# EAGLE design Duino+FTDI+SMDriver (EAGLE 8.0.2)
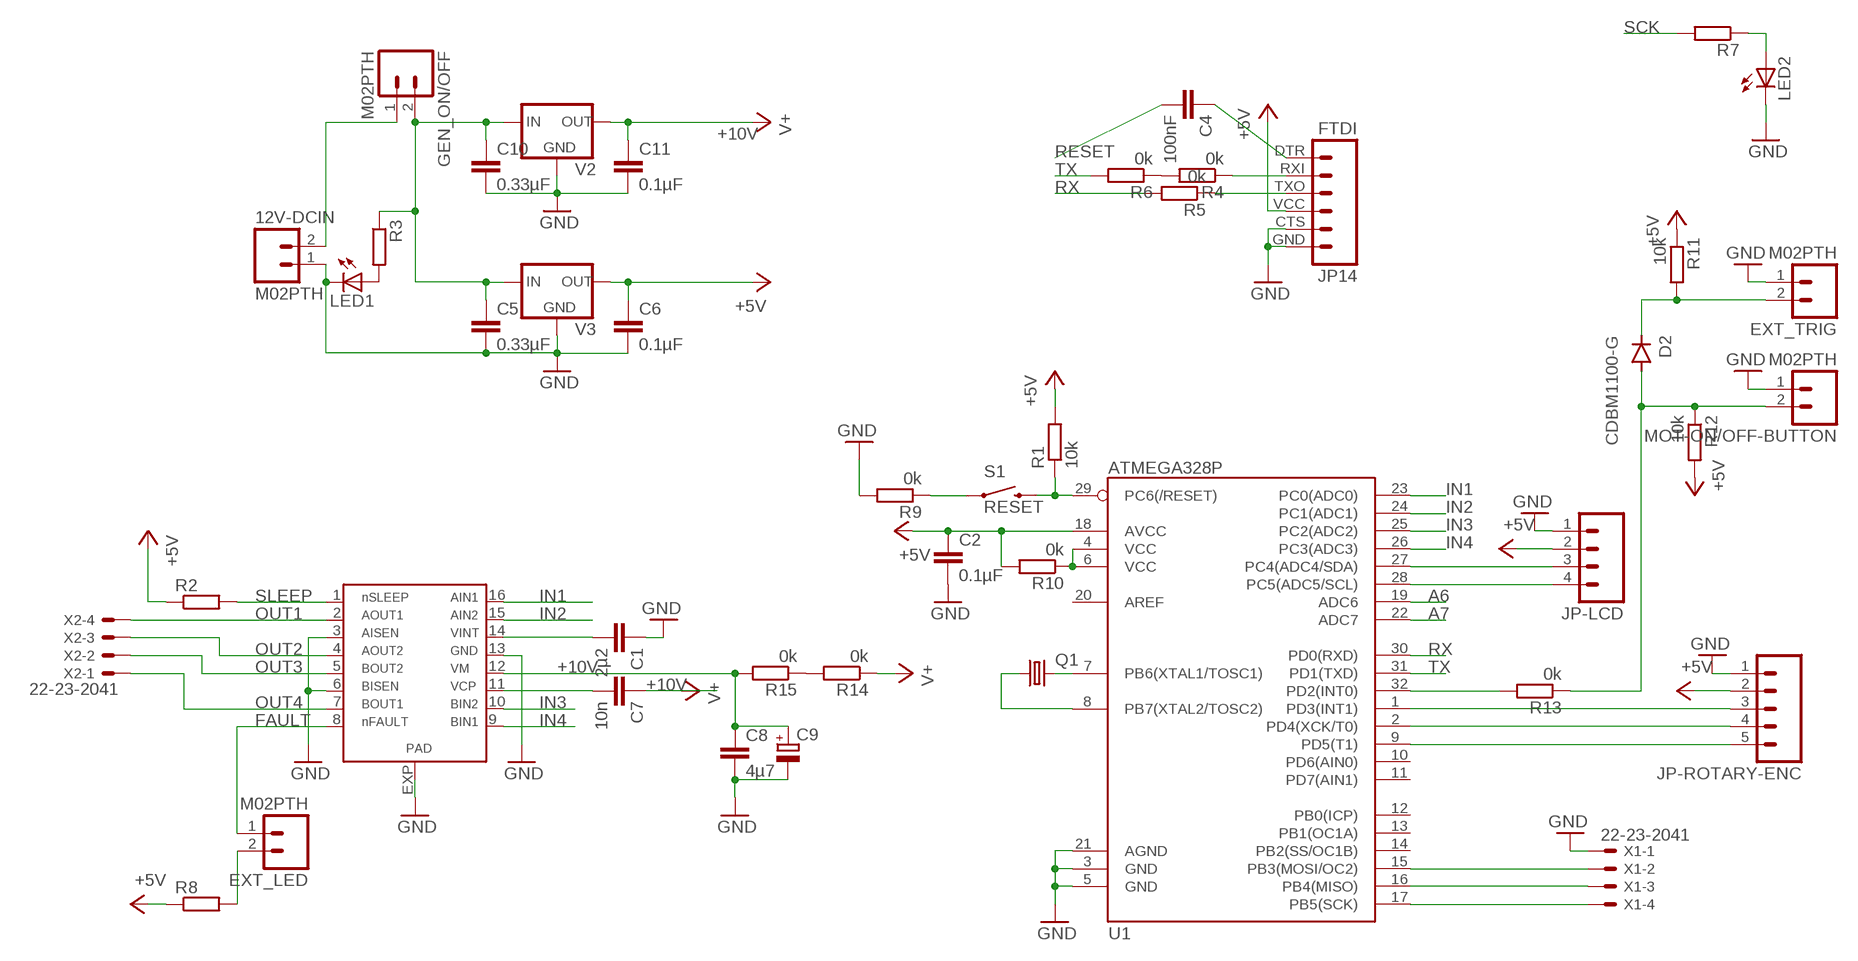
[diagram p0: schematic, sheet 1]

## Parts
12V-DCIN  M02PTH  [1X02]
C1  2µ2  C-EUC1206  [C1206]
C2  0.1µF  C-EUC1206  [C1206]
C4  100nF  C-EUC1206  [C1206]
C5  0.33µF  C-EUC1206  [C1206]
C6  0.1µF  C-EUC1206  [C1206]
C7  10n  C-EUC1206  [C1206]
C8  4µ7  C-EUC1206  [C1206]
C9  CPOL-EU153CLV-0605  [153CLV-0605]
C10  0.33µF  C-EUC1206  [C1206]
C11  0.1µF  C-EUC1206  [C1206]
D2  CDBM1100-G  [MINI-SMA]
EXT_LED  M02PTH  [1X02]
EXT_TRIG  M02PTH  [1X02]
GEN_ON/OFF  M02PTH  [1X02]
IC1  DRV8833  [HTSSOP16PWP]
JP14  FTDI  FTDI_BASICPTH  [FTDI_BASIC]
JP-LCD  M04PTH  [1X04]
JP-ROTARY-ENC  M05PTH  [1X05]
LED1  LEDSMT1206  [1206]
LED2  LEDSMT1206  [1206]
MOT-ON/OFF-BUTTON  M02PTH  [1X02]
Q1  CRYSTALSM49  [SM49]
R1  10k  R-EU_R1206  [R1206]
R2  R-EU_R1206  [R1206]
R3  R-EU_R1206  [R1206]
R4  0k  R-EU_R1206  [R1206]
R5  0k  R-EU_R1206  [R1206]
R6  0k  R-EU_R1206  [R1206]
R7  R-EU_R1206  [R1206]
R8  R-EU_R1206  [R1206]
R9  0k  R-EU_R1206  [R1206]
R10  0k  R-EU_R1206  [R1206]
R11  10k  R-EU_R1206  [R1206]
R12  10k  R-EU_R1206  [R1206]
R13  0k  R-EU_R1206  [R1206]
R14  0k  R-EU_R1206  [R1206]
R15  0k  R-EU_R1206  [R1206]
S1  RESET  SWITCH-MOMENTARY-2-SMD-1101NE  [TACTILE-SWITCH-1101NE]
U1  ATMEGA328P  ATMEGA328_SMT  [TQFP32-08]
V2  UA78XX  [D2PACK]
V3  UA78MXX  [DPACK]
X1  22-23-2041  [22-23-2041]
X2  22-23-2041  [22-23-2041]

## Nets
+5V: C2.1 C6.1 JP14.VCC JP-LCD.2 JP-ROTARY-ENC.2 R1.2 R2.1 R8.1 R10.1 R10.2 R11.1 R12.2 U1.4(VCC) U1.6(VCC) U1.18(AVCC) V3.OUT
+10V: C7.1 C8.1 C9.+ C11.1 IC1.12 R14.1 R15.2 V2.OUT ; supply symbol labelled V+
A4: JP-LCD.3 U1.27(PC4(ADC4/SDA))
A5: JP-LCD.4 U1.28(PC5(ADC5/SCL))
A6: U1.19(ADC6)
A7: U1.22(ADC7)
FAULT: EXT_LED.1 IC1.8
GND: 12V-DCIN.1 C1.1 C2.2 C5.2 C6.2 C8.2 C9.- C10.2 C11.2 EXT_TRIG.1 IC1.3 IC1.6 IC1.13 IC1.EXP JP14.CTS JP14.GND JP-LCD.1 JP-ROTARY-ENC.1 LED1.C LED2.C MOT-ON/OFF-BUTTON.1 R9.1 R9.2 S1.1 U1.3(GND) U1.5(GND) U1.21(AGND) V2.CASE(GND) V2.GND V3.CASE(GND) X1.1
IN1: IC1.16 U1.23(PC0(ADC0))
IN2: IC1.15 U1.24(PC1(ADC1))
IN3: IC1.10 U1.25(PC2(ADC2))
IN4: IC1.9 U1.26(PC3(ADC3))
N$1: Q1.2 U1.7(PB6(XTAL1/TOSC1))
N$2: Q1.1 U1.8(PB7(XTAL2/TOSC2))
N$3: JP-ROTARY-ENC.3 U1.1(PD3(INT1))
N$4: 12V-DCIN.2 GEN_ON/OFF.1
N$5: C4.1 JP14.DTR
N$6: JP14.RXI R4.1
N$7: JP14.TXO R5.1
N$8: R4.2 R6.1
N$9: LED2.A R7.1
N$10: R13.2 U1.32(PD2(INT0))
N$11: D2.KATHODE EXT_TRIG.2 R11.2
N$13: R14.2 R15.1
N$14: LED1.A R3.2
N$15: D2.ANODE MOT-ON/OFF-BUTTON.2 R12.1 R13.1
N$17: U1.16(PB4(MISO)) X1.3
N$18: U1.15(PB3(MOSI/OC2)) X1.2
N$19: JP-ROTARY-ENC.4 U1.2(PD4(XCK/T0))
N$20: JP-ROTARY-ENC.5 U1.9(PD5(T1))
N$22: C1.2 IC1.14
N$23: C7.2 IC1.11
N$25: EXT_LED.2 R8.2
N$26: C5.1 C10.1 GEN_ON/OFF.2 R3.1 V2.IN V3.IN
OUT1: IC1.2 X2.4
OUT2: IC1.4 X2.3
OUT3: IC1.5 X2.2
OUT4: IC1.7 X2.1
RESET: C4.2 R1.1 S1.2 U1.29(PC6(/RESET))
RX: R5.2 U1.30(PD0(RXD))
SCK: R7.2 U1.17(PB5(SCK)) X1.4
SLEEP: IC1.1 R2.2
TX: R6.2 U1.31(PD1(TXD))
Unconnected: U1.10(PD6(AIN0)) U1.11(PD7(AIN1)) U1.12(PB0(ICP)) U1.13(PB1(OC1A)) U1.14(PB2(SS/OC1B)) U1.20(AREF)

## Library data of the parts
12V-DCIN EXT_LED EXT_TRIG GEN_ON/OFF MOT-ON/OFF-BUTTON = SparkFun-Connectors:M02: Standard 2-pin 0.1" header. Use with
C1 C2 C4-C8 C10 C11 = rcl:C-EU: CAPACITOR, European symbol
C9 = rcl:CPOL-EU: POLARIZED CAPACITOR, European symbol
D2 = fab:CDBM1100-G: Diode schottky 100V 1A mini-SMA as found in the fablab inventory
IC1 = 1Axel:DRV8833
JP14 = SparkFun-Connectors:FTDI_BASIC: FTDI Basic header with labels
JP-LCD = SparkFun-Connectors:M04: Header 4 Standard 4-pin 0.1" header. Use with straight break away headers (SKU : PRT-00116), right angle break away headers (PRT-00553), swiss pins (PRT-00743), machine pins (PRT-00117), and female headers (PRT-00115). Molex polarized connector foot print use with SKU : PRT-08231 with associated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
JP-ROTARY-ENC = SparkFun-Connectors:M05: Header 5 Standard 5-pin 0.1" header. Use with straight break away headers (SKU : PRT-00116), right angle break away headers (PRT-00553), swiss pins (PRT-00743), machine pins (PRT-00117), and female headers (PRT-00115). Molex polarized connector foot print use with SKU : PRT-08230 with associated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
LED1 LED2 = led:LED: LED
Q1 = crystal:CRYSTAL: CRYSTAL; OC_FARNELL: unknown; OC_NEWARK: unknown
R1-R15 = rcl:R-EU_: RESISTOR, European symbol
S1 = SparkFun-Electromechanical:SWITCH-MOMENTARY-2: Various NO switches- pushbuttons, reed, etc
U1 = SparkFun-DigitalIC:ATMEGA328_SMT: 32-Pin Atmega328 part Commonly used on Arduino compatible boards Available in QFP and QFN packages TQFP is IC-09069 QFN is non-stock; PROD_ID: IC-09069
V2 = Power:UA78XX
V3 = Power:UA78MXX
X1 X2 = con-molex:22-23-2041: .100" (2.54mm) Center Header - 4 Pin; MF: MOLEX; MPN: 22-23-2041; OC_FARNELL: 1462920; OC_NEWARK: 38C0355

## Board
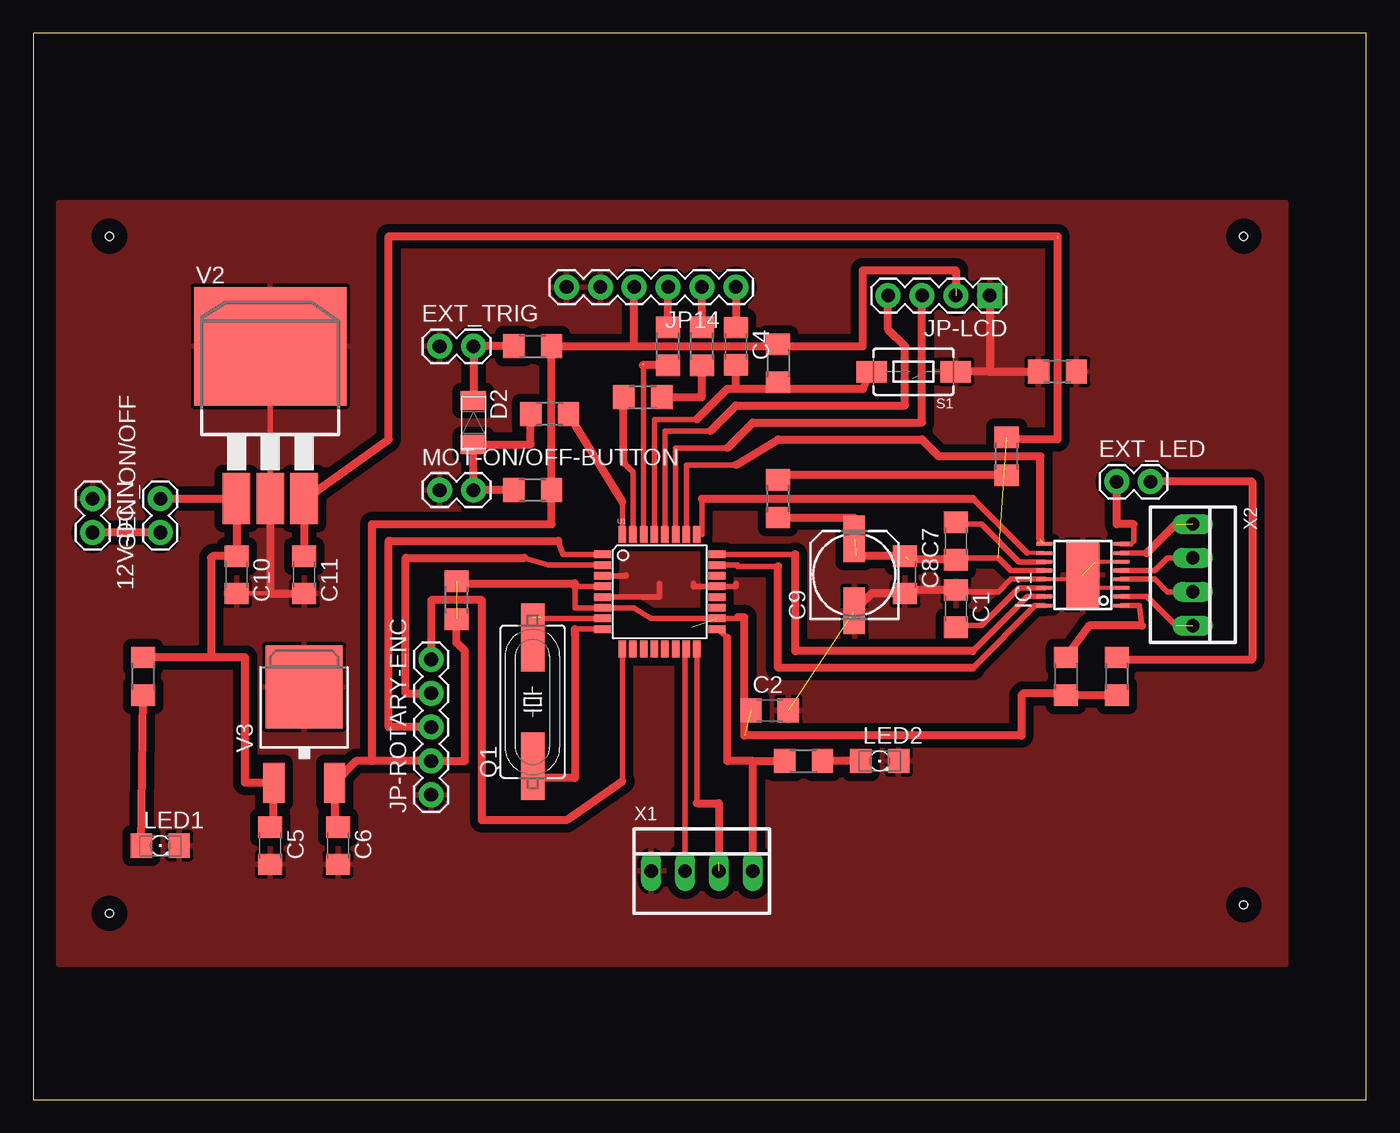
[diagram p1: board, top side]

Size 100 x 80 mm. Coordinates in mm from the lower left corner, seen from the top.
Outline: 0,0 100,0 100,80 0,80 0,0
Copper layers (1*16): Top 0.035mm / dielectric 1.5mm / Bottom 0.035mm
Design rules "default": minimum track width 10mil, minimum drill 24mil, track to track 8mil, track to pad 8mil, pad to pad 8mil, via to via 8mil, smd to smd 8mil, copper to edge 40mil, drill to drill 8mil, minimum pad ring 10mil, minimum via ring 8mil, stop-mask expansion 4mil, vias tented up to drill 0mil, thermal gap 10mil
Holes 0.6 mm at 5.71,13.97 5.71,64.77 90.81,64.77 90.81,14.61

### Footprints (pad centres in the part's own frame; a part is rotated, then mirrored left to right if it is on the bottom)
1X02 = drill 1.016 pad 1.88: 1 0,0; 2 2.54,0
C1206 = smd 1.6 x 1.8: 1 -1.4,0; 2 1.4,0
153CLV-0605 = smd 3.5 x 1.6: + 2.7,0; - -2.7,0
MINI-SMA = smd 1.4 x 1.9: ANODE 1.65,0; KATHODE -1.65,0
HTSSOP16PWP = smd 0.27 x 1.2: 1 -3.588,-2.9; 2 -2.895,-2.9; 3 -2.245,-2.9; 4 -1.595,-2.9; 5 -0.945,-2.9; 6 -0.295,-2.9; 7 0.355,-2.9; 8 1.048,-2.9; 9 1.048,2.9; 10 0.355,2.9; 11 -0.295,2.9; 12 -0.945,2.9; 13 -1.595,2.9; 14 -2.245,2.9; 15 -2.895,2.9; 16 -3.588,2.9 | smd 5.08 x 2.46: EXP -1.27,0
FTDI_BASIC = drill 1.016 pad 1.88: CTS 10.16,0; DTR 0,0; GND 12.7,0; RXI 2.54,0; TXO 5.08,0; VCC 7.62,0
1X04 = drill 1.016 pad 1.88 square: 1 0,0 | drill 1.016 pad 1.88: 2 2.54,0; 3 5.08,0; 4 7.62,0
1X05 = drill 1.016 pad 1.88: 1 0,0; 2 2.54,0; 3 5.08,0; 4 7.62,0; 5 10.16,0
1206 = smd 1.6 x 1.803: A -1.422,0; C 1.422,0
SM49 = smd 5.08 x 1.778: 1 -4.826,0; 2 4.826,0
R1206 = smd 1.6 x 1.803: 1 -1.422,0; 2 1.422,0
TACTILE-SWITCH-1101NE = smd 2.3 x 1.6: 1 -3.15,0; 2 3.15,0
TQFP32-08 = smd 1.27 x 0.559: 1 -4.293,2.8; 2 -4.293,2; 3 -4.293,1.2; 4 -4.293,0.4; 5 -4.293,-0.4; 6 -4.293,-1.2; 7 -4.293,-2; 8 -4.293,-2.8; 17 4.293,-2.8; 18 4.293,-2; 19 4.293,-1.2; 20 4.293,-0.4; 21 4.293,0.4; 22 4.293,1.2; 23 4.293,2; 24 4.293,2.8 | smd 0.559 x 1.27: 9 -2.8,-4.293; 10 -2,-4.293; 11 -1.2,-4.293; 12 -0.4,-4.293; 13 0.4,-4.293; 14 1.2,-4.293; 15 2,-4.293; 16 2.8,-4.293; 25 2.8,4.293; 26 2,4.293; 27 1.2,4.293; 28 0.4,4.293; 29 -0.4,4.293; 30 -1.2,4.293; 31 -2,4.293; 32 -2.8,4.293
D2PACK = smd 11.43 x 8.89: CASE 3.81,6.35 | smd 2.083 x 3.81: GND 3.81,-5.08; IN 1.27,-5.08; OUT 6.35,-5.08
DPACK = smd 5.8 x 6.2: CASE 0,2.38 | smd 1.6 x 3: IN -2.28,-4.8; OUT 2.28,-4.8
22-23-2041 = drill 1 long: 1 -3.81,0; 2 -1.27,0; 3 1.27,0; 4 3.81,0

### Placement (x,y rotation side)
12V-DCIN  4.45,45.09 270 top
C1  69.22,36.83 270 top
C2  55.24,29.21 0 top
C4  52.7,56.52 270 top
C5  17.78,19.05 270 top
C6  22.86,19.05 270 top
C7  69.22,41.91 90 top
C8  65.41,39.37 270 top
C9  61.59,39.37 90 top
C10  15.24,39.37 270 top
C11  20.32,39.37 270 top
D2  33.02,50.8 270 top
EXT_LED  81.28,46.35 0 top
EXT_TRIG  30.48,56.52 0 top
GEN_ON/OFF  9.53,42.55 90 top
IC1  78.74,40.64 90 top
JP14  52.7,60.96 180 top
JP-LCD  71.75,60.33 180 top
JP-ROTARY-ENC  29.84,22.86 90 top
LED1  9.53,19.05 0 top
LED2  63.5,25.4 0 top
MOT-ON/OFF-BUTTON  30.48,45.72 0 top
Q1  37.47,29.84 90 top
R1  55.88,55.24 90 top
R2  77.47,31.75 90 top
R3  8.26,31.75 270 top
R4  50.16,56.52 270 top
R5  47.62,56.52 270 top
R6  45.72,52.7 180 top
R7  57.78,25.4 180 top
R8  81.28,31.75 90 top
R9  76.83,54.61 0 top
R10  31.75,37.47 270 top
R11  37.47,56.52 180 top
R12  37.47,45.72 0 top
R13  38.73,51.44 0 top
R14  73.03,48.26 270 top
R15  55.88,45.09 270 top
S1  66.04,54.61 180 top
U1  46.99,38.1 0 top
V2  13.97,50.16 0 top
V3  20.32,28.57 0 top
X1  50.16,17.14 0 top
X2  87,39.37 270 top

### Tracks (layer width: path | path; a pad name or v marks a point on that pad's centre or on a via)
+5V  (5 unrouted)
  Top 0.305: 55.88,56.52 R1.2
  Top 0.406: 22.6,20.71 C6.1 | 52.84,36.2 52.84,36.1 U1.18 46.35,36.1 45.09,36.9 U1.6 40.64,36.9 40.64,38.5 U1.4
  Top 0.61: R8.1 R2.1 77.32,30.48 74.3,30.48 74.14,30.33 74.14,27.3 53.34,27.3 53.34,36.2 52.84,36.2 | 25.4,25.4 JP-ROTARY-ENC.2 32.38,25.4 32.38,33.66 31.75,34.29 R10.2 | 25.4,25.4 25.4,43.18 38.89,43.18 R12.2 R11.1 45.09,56.52 | 45.09,56.52 JP14.VCC | 45.09,56.52 55.88,56.52 62.23,56.52 62.23,62.23 69.22,62.23 69.22,60.85 | 40.64,38.5 40.64,38.73 31.75,38.73 | 22.6,20.71 V3.OUT 24.23,25.4 25.4,25.4
+10V  (4 unrouted)
  Top 0.305: C7.1 69.34,40.64 | C11.1 20.45,45.09 | 61.73,40.77 61.59,40.64
  Top 0.406: 69.34,40.64 72.39,40.64 73.33,39.7 IC1.12
  Top 0.61: C7.1 65.67,40.51 | V2.OUT C11.1 | 20.45,45.09 26.67,49.53 26.67,64.77 76.83,64.77 | 76.83,64.61 76.83,49.53 74.3,49.53 R14.1 | C8.1 61.73,40.77 | R15.2 61.59,43.66 C9.+
A4
  Top 0.406: 52.07,48.9 48.19,48.9 U1.27
  Top 0.61: JP-LCD.3 66.67,50.8 53.98,50.8 52.07,48.9
A5
  Top 0.406: 50.8,50.16 47.39,50.16 U1.28
  Top 0.61: 50.8,50.16 52.7,52.07 65.41,52.07 65.41,56.52 64.14,57.78 JP-LCD.4
FAULT
  Top 0.305: 82.33,41.69 82.55,41.91
  Top 0.406: IC1.8 82.33,41.69 | 82.55,41.91 82.55,43.18
  Top 0.61: 82.55,43.18 81.28,43.18 EXT_LED.1
GND  (2 unrouted)
  Top 0.305: 69.34,38.1 C1.1 | IC1.13 78.42,39.05 IC1.EXP | IC1.3 79.03,38.4 78.74,38.1 | IC1.6 79.67,40.34 79.38,40.64 | 65.67,38.23 C8.2 | 17.78,37.97 C10.2
  Top 0.406: 17.78,55.88 V2.GND | IC1.13 73.33,39.05 72.39,38.1 69.34,38.1 | 49.53,38.73 49.53,38.5 U1.21 52.7,38.5 52.7,38.73 | U1.3 44.45,39.3 44.45,39.37 | U1.5 46.99,37.7 46.99,38.73
  Top 0.61: C1.1 65.67,38.23 | C8.2 62.9,37.97 C9.- | C11.2 17.78,37.97 V2.GND | 71.75,54.61 S1.1 | 71.75,54.61 R9.1 | JP-LCD.1 71.75,54.61
  pour Top (isolate 0.61): 93.98,10.16 1.91,10.16 1.91,67.31 93.98,67.31
IN1
  Top 0.406: IC1.16 75.15,37.05 70.48,32.38 | 55.88,40.01 52.84,40.01 52.84,40.1 U1.23
  Top 0.61: 70.48,32.38 55.88,32.38 55.88,40.01
IN2
  Top 0.406: IC1.15 74.58,37.74 70.48,33.66 | U1.24 57.15,40.9
  Top 0.61: 70.48,33.66 57.15,33.66 57.15,40.9
IN3
  Top 0.305: IC1.10 74.58,40.99
  Top 0.406: 74.58,40.99 70.48,45.09 | U1.25 50.16,42.39 50.16,45.09
  Top 0.61: 50.16,45.09 70.48,45.09
IN4  (1 unrouted)
  Top 0.305: 49.16,42.56 U1.26
  Top 0.406: 52.7,47.62 48.99,47.62 U1.26
  Top 0.61: 52.7,47.62 55.88,49.53 66.67,49.53 67.94,48.26 75.56,48.26 75.56,41.96
N$1  (1 unrouted)
  Top 0.305: 38.2,36.1 38.1,36.2 38.1,32.38
  Top 0.406: U1.7 37.47,36.1 37.47,36.2 Q1.2
N$2
  Top 0.305: 38.1,24.13 Q1.1
  Top 0.406: U1.8 40.64,35.3 40.64,34.92
  Top 0.61: 40.64,35.3 40.64,34.92 40.64,24.13 38.1,24.13
N$3
  Top 0.406: 39.37,41.91 39.74,40.9 U1.1
  Top 0.61: JP-ROTARY-ENC.3 26.67,27.94 26.67,41.91 39.37,41.91
N$4
  Top 0.61: GEN_ON/OFF.1 12V-DCIN.2
N$5
  Top 0.61: JP14.DTR C4.1
N$6
  Top 0.61: R4.1 JP14.RXI
N$7
  Top 0.61: R5.1 JP14.TXO
N$8
  Top 0.61: R6.1 50.16,52.7 R4.2
N$9
  Top 0.61: LED2.A R7.1
N$10
  Top 0.406: U1.32 44.19,44.86
  Top 0.61: 44.19,44.86 R13.2
N$11
  Top 0.61: R11.2 EXT_TRIG.2 D2.KATHODE
N$13
  Top 0.61: R14.2 55.88,46.84 R15.1
N$14
  Top 0.61: LED1.A R3.2
N$15
  Top 0.406: 36.2,45.72 R12.1
  Top 0.61: R12.1 MOT-ON/OFF-BUTTON.2 D2.ANODE 37.31,49.15 R13.1
N$17  (1 unrouted)
  Top 0.406: U1.16 49.79,22.23
  Top 0.61: 49.79,22.23 51.44,22.23 51.44,17.78
N$18
  Top 0.305: 48.9,33.71 U1.15
  Top 0.406: 48.9,33.81 U1.15 48.9,33.81 | 48.9,33.81 X1.2
N$19
  Top 0.406: 36.83,40.64 38.64,40.1 U1.2
  Top 0.61: JP-ROTARY-ENC.4 27.94,30.48 27.94,40.64 36.83,40.64
N$20
  Top 0.406: U1.9 44.19,23.87
  Top 0.61: 44.19,23.87 40.01,20.95 33.66,20.95 33.66,37.47 29.84,37.47 JP-ROTARY-ENC.5
N$22
  Top 0.305: 69.34,35.56 C1.2
  Top 0.406: IC1.14 73.95,38.4 71.12,35.56 69.34,35.56
N$23
  Top 0.305: 69.34,43.18 C7.2
  Top 0.406: IC1.11 73.95,40.34 71.12,43.18 69.34,43.18
N$25
  Top 0.406: 81.28,33.02 R8.2
  Top 0.61: EXT_LED.2 91.44,46.35 91.44,33.02 81.28,33.02
N$26
  Top 0.305: 15.24,40.64 C10.1
  Top 0.406: 18.04,20.71 C5.1 | 13.46,40.77 13.34,40.64
  Top 0.61: GEN_ON/OFF.2 V2.IN C10.1 13.46,40.77 | 13.34,33.17 R3.1 | 13.34,33.17 15.88,33.17 15.88,23.77 V3.IN 18.04,20.71 | 13.34,40.64 13.34,33.17
OUT1  (1 unrouted)
  Top 0.406: IC1.2 83.54,37.74 85.72,35.56
OUT2
  Top 0.406: IC1.4 84.14,39.05 85.09,38.1 X2.3
OUT3
  Top 0.406: IC1.5 84.14,39.7 85.09,40.64 X2.2
OUT4  (1 unrouted)
  Top 0.406: IC1.7 83.54,40.99
  Top 0.61: 83.54,40.99 85.72,43.18
RESET
  Top 0.406: 49.77,51.03 46.59,51.03 U1.29
  Top 0.61: 49.77,51.03 52.07,53.34 52.7,53.34 | 52.7,53.34 C4.2 | 52.7,53.34 55.88,53.34 | 55.88,53.34 R1.1 | 55.88,53.34 62.26,53.34 S1.2
RX  (1 unrouted)
  Top 0.406: U1.30 45.79,55.16
  Top 0.61: R5.2 45.72,55.09
SCK
  Top 0.406: U1.17 52.07,34.66
  Top 0.61: 52.07,34.66 52.07,25.4 53.98,25.4 | 53.98,25.4 R7.2 | X1.4 53.98,25.4
SLEEP
  Top 0.406: IC1.1 82.96,37.05 83.19,35.56
  Top 0.61: 83.19,35.56 79.22,35.56 R2.2
TX
  Top 0.406: 44.3,47.78 44.99,47.09 U1.31
  Top 0.61: 44.3,47.78 R6.2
